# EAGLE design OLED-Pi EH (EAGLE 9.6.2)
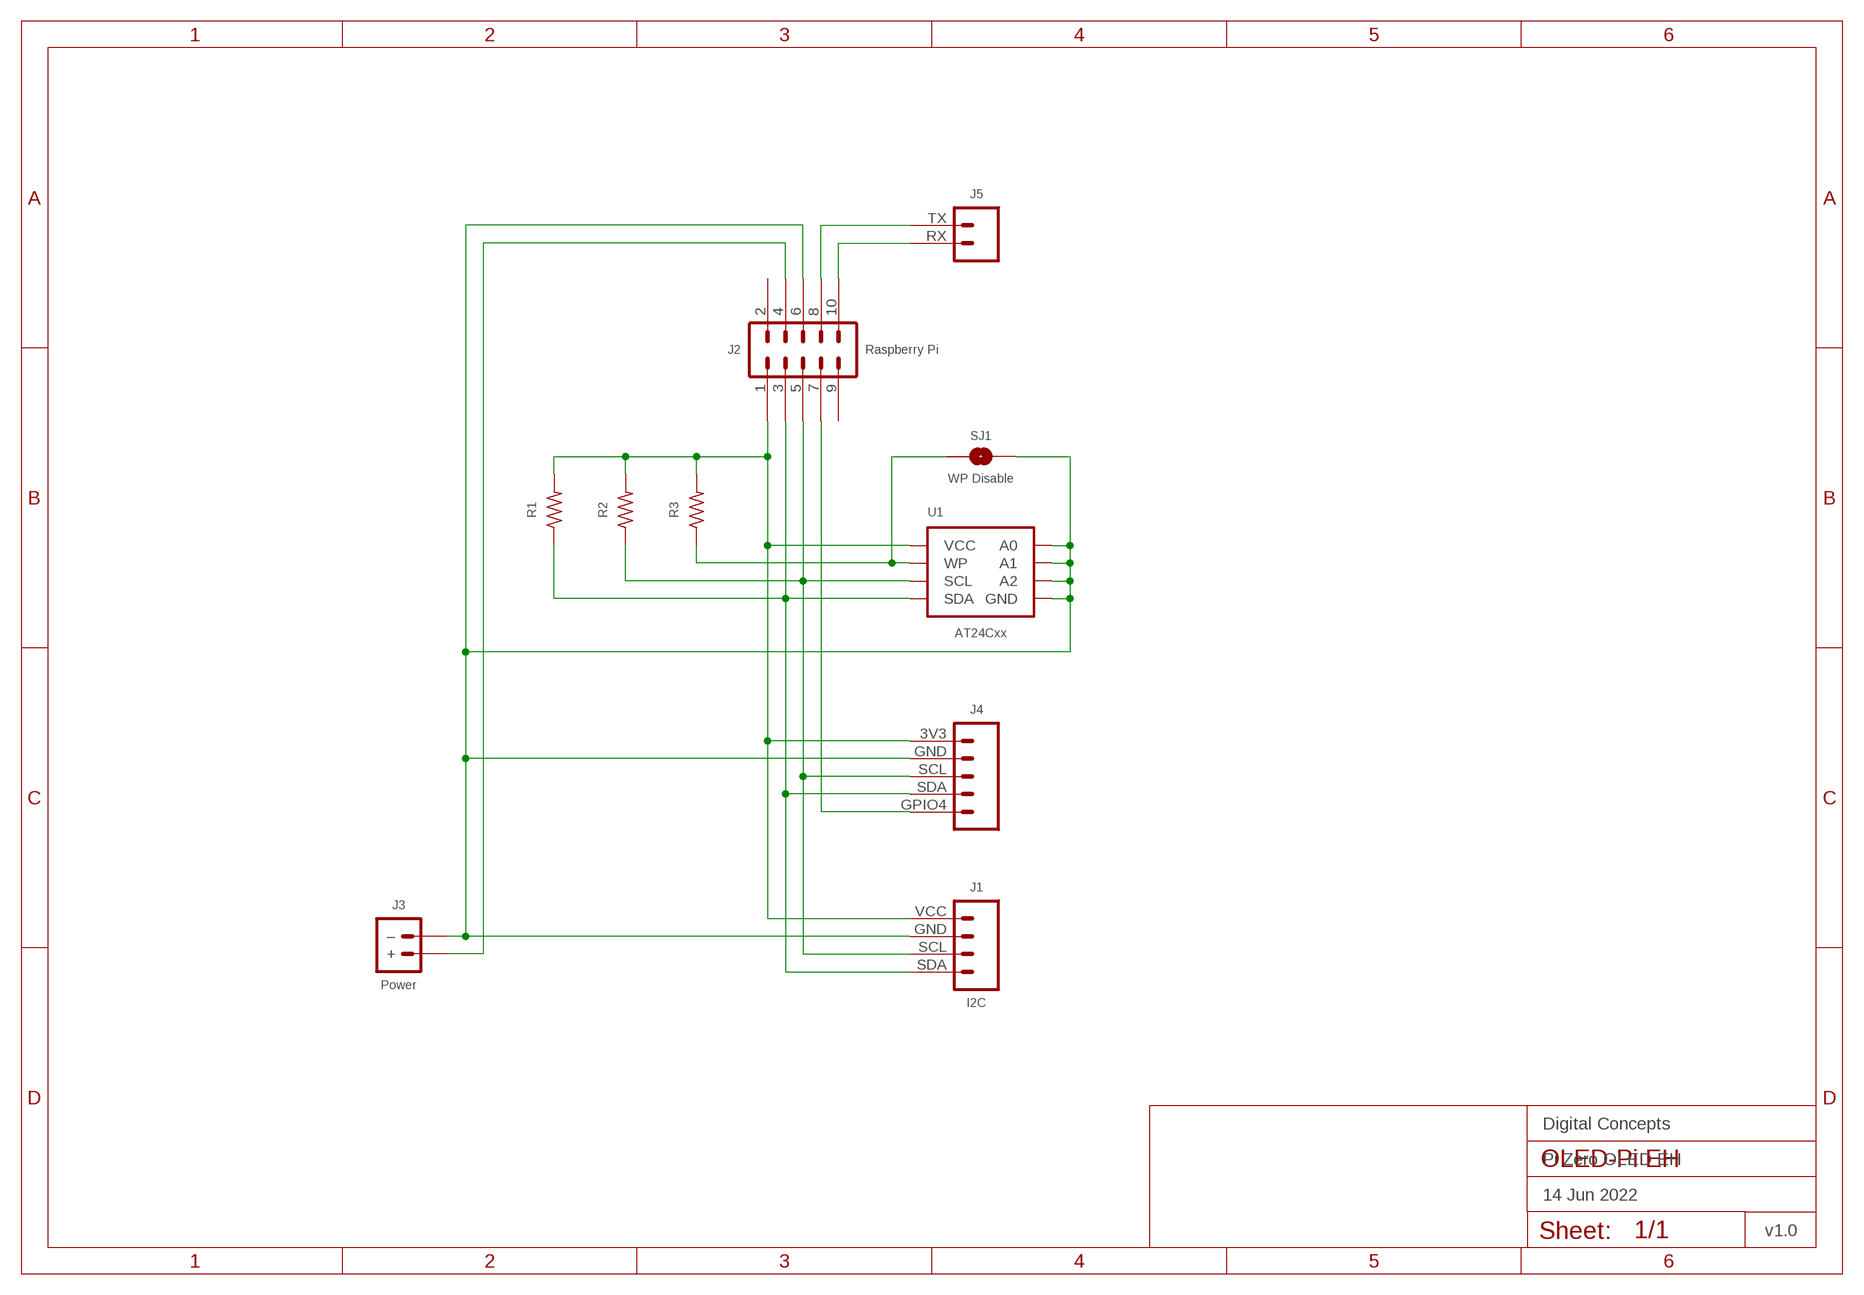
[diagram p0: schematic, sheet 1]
FRAME1 (FRAME-A4L-LOC): DATE: 14 Jun 2022; OWNER: Digital Concepts; TITLE: Pi Zero OLED EH; VERSION: v1.0

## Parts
J1  I2C  HEADER-1X4-I2C  [CONN_04-I2C]
J2  Raspberry Pi  HEADER-2X5-PI-1  [CONN_2X5-PI-1]
J3  Power  JST-PH2.0-2-HORIZONTAL-POWERJST-PTH-2  [JST-PH2.0-2-HORIZONTAL-POWER]
J4  JST-PH2.0-5-HORIZONTAL-OLED-PI  [JST-PH2.0-5-HORIZONTAL-OLED-PI]
J5  JST-PH2.0-2-HORIZONTAL-TX-RXJST-PTH-2  [JST-PH2.0-2-HORIZONTAL=TX-RX]
R1  RESISTORR0805  [R0805]
R2  RESISTORR0805  [R0805]
R3  RESISTORR0805  [R0805]
SJ1  WP Disable  SJ  [SJ]
U1  AT24Cxx  AT24CXX-EEPROM  [SOP-8]

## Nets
GND: J1.GND J2.6 J3.-(–) J4.GND SJ1.2 U1.P$1(A0) U1.P$2(A1) U1.P$3(A2) U1.P$4(GND)
N$2: J2.4 J3.+
N$4: J1.SDA J2.3 J4.SDA R1.1 U1.P$5(SDA)
N$5: J1.SCL J2.5 J4.SCL R2.1 U1.P$6(SCL)
N$6: J2.7 J4.GPIO4
N$7: J2.10 J5.RX
N$8: J2.8 J5.TX
N$9: R3.1 SJ1.1 U1.P$7(WP)
VCC: J1.VCC J2.1 J4.3V3 R1.2 R2.2 R3.2 U1.P$8(VCC)
Unconnected: J2.2 J2.9

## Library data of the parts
J1 = digitalconcepts:HEADER-1X4-I2C: I2C Interface [Pin 1 Vcc] 4-Pin Header
J2 = digitalconcepts:HEADER-2X5-PI-1: Ras-Pi 2x5 PTH Header Rapsberry Pi, starting at Pin 1
J3 = digitalconcepts:JST-PH2.0-2-HORIZONTAL-POWER: PH2.0 2P Right Angle PCB Connector; PROD_ID: CONN-09863; SKU: PRT-09914
J4 = digitalconcepts:JST-PH2.0-5-HORIZONTAL-OLED-PI: PH2.0 5P OLED-Pi Horizontal Connector
J5 = digitalconcepts:JST-PH2.0-2-HORIZONTAL-TX-RX: PH2.0 2P Right Angle PCB Connector with Tx/Rx Pin Labels; PROD_ID: CONN-09863; SKU: PRT-09914
R1-R3 = digitalconcepts:RESISTOR: Resistor; SPICEPREFIX: R
SJ1 = digitalconcepts:SJ: Solder Jumper
U1 = digitalconcepts:AT24CXX-EEPROM: AT24Cxx EEPROM SOP-8

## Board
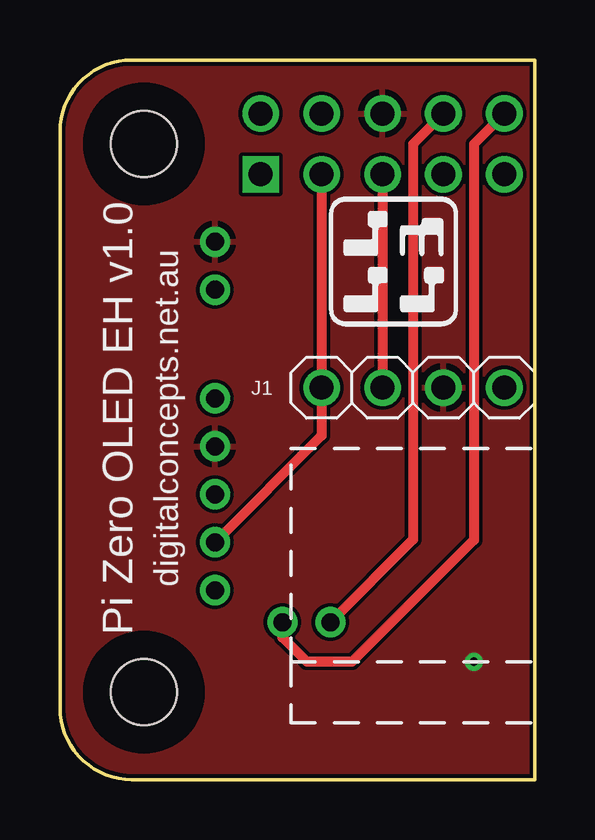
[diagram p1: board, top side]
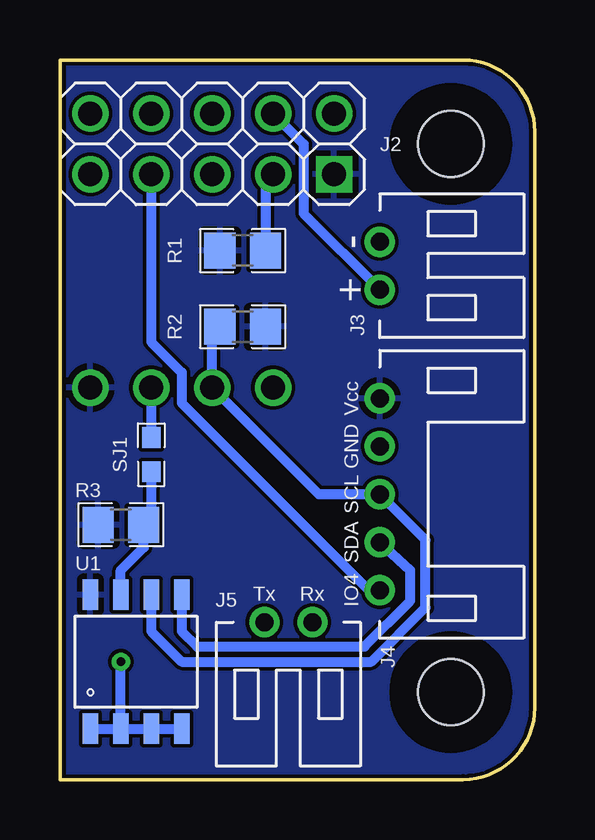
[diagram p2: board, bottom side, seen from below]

Size 19.8 x 30 mm. Coordinates in mm from the lower left corner, seen from the top.
Outline: 19.8,30 19.8,0 2.99,0 arc-90 0,2.99 0,27.01 arc-90 2.99,30 19.8,30
Copper layers (1*16): Top 0.035mm / dielectric 1.5mm / Bottom 0.035mm
Design rules "default *": minimum track width 6mil, minimum drill 0.35mm, track to track 6mil, track to pad 6mil, pad to pad 6mil, via to via 6mil, smd to smd 6mil, copper to edge 6mil, drill to drill 6mil, minimum pad ring 10mil, minimum via ring 8mil, stop-mask expansion 4mil, vias tented up to drill 0mil, thermal gap 10mil
Holes 2.75 mm at 3.5,26.5 3.5,3.64

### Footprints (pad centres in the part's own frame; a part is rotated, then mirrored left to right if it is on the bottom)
CONN_04-I2C = drill 1 pad 1.524: GND 2.54,0; SCL 5.08,0; SDA 7.62,0; VCC 0,0
CONN_2X5-PI-1 = drill 1 pad 1.524 square: 1 0,0 | drill 1 pad 1.524: 2 0,2.54; 3 2.54,0; 4 2.54,2.54; 5 5.08,0; 6 5.08,2.54; 7 7.62,0; 8 7.62,2.54; 9 10.16,0; 10 10.16,2.54
JST-PH2.0-2-HORIZONTAL-POWER = drill 0.75: + 1,0; - -1,0
JST-PH2.0-5-HORIZONTAL-OLED-PI = drill 0.75: 3V3 4,0; GND 2,0; GPIO4 -4,0; SCL 0,0; SDA -2,0
JST-PH2.0-2-HORIZONTAL=TX-RX = drill 0.75: RX -1,0; TX 1,0
R0805 = smd 1.3 x 1.5: 1 -0.95,0; 2 0.95,0
SJ = smd 0.864 x 0.762: 1 -0.711,0; 2 0.711,0
SOP-8 = smd 0.635 x 1.27: P$1 -1.905,-2.794; P$2 -0.635,-2.794; P$3 0.635,-2.794; P$4 1.905,-2.794; P$5 1.905,2.794; P$6 0.635,2.794; P$7 -0.635,2.794; P$8 -1.905,2.794

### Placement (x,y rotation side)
J1  18.53,16.34 180 top
J2  8.37,25.23 0 top
J3  6.47,21.42 270 bottom
J4  6.47,11.89 90 bottom
J5  10.28,6.56 180 bottom
R1  12.18,22.05 180 bottom
R2  12.18,18.88 0 bottom
R3  17.26,10.62 180 bottom
SJ1  15.99,13.55 90 bottom
U1  16.63,4.91 0 bottom

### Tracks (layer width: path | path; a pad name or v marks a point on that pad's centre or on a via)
$X1
  cutout Top: 3.5,6.18 arc180 3.5,1.1 arc180
$X2
  cutout Top: 3.5,29.04 arc180 3.5,23.96 arc180
$X3
  cutout Bottom: 3.5,6.18 arc180 3.5,1.1 arc180
$X4
  cutout Bottom: 3.5,29.04 arc180 3.5,23.96 arc180
GND  (via drill 0.35)
  Bottom 0.406: U1.P$4 U1.P$3 U1.P$2 | U1.P$1 U1.P$2 | J1.GND SJ1.2 | U1.P$2 v17.26,4.91
  pour Top: 21.07,31.58 -1.15,31.58 -1.15,-1.44 21.07,-1.44
N$2
  Bottom 0.406: J2.4 9.64,26.5 9.64,23.59 J3.+
N$4
  Top 0.406: J2.3 J1.SDA 10.91,14.34 J4.SDA
  Bottom 0.406: U1.P$5 14.72,6.18 14.09,5.54 7.1,5.54 5.2,7.45 5.2,8.72 J4.SDA | J2.3 11.23,24.91 R1.1
N$5
  Top 0.406: J2.5 J1.SCL
  Bottom 0.406: U1.P$6 15.99,6.18 14.72,4.91 6.82,4.91 4.56,7.17 4.56,9.99 J4.SCL 9.01,11.89 J1.SCL 13.45,18.56 R2.1
N$6
  Bottom 0.406: J4.GPIO4 6.91,7.89 14.72,15.7 14.72,16.97 15.99,18.24 J2.7
N$7
  Top 0.406: J2.10 17.26,26.5 17.26,9.99 12.18,4.91 10.29,4.91 9.28,5.93 J5.RX
N$8
  Top 0.406: J2.8 14.72,26.5 14.72,10.01 J5.TX
N$9
  Bottom 0.406: U1.P$7 17.26,8.72 16.31,9.67 R3.1 15.99,10.94 SJ1.1
VCC
  pour Bottom: 20.44,30.94 -0.52,30.94 -0.52,-0.81 20.44,-0.81

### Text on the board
tPlace: Pi Zero OLED EH v1.0 | digitalconcepts.net.au
bNames: Vcc | GND | SCL | SDA | IO4 | Rx | Tx
tValues: SDA | SCL | GND | VCC
bValues: 5V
